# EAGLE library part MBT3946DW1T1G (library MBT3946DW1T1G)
Source: Datasheet
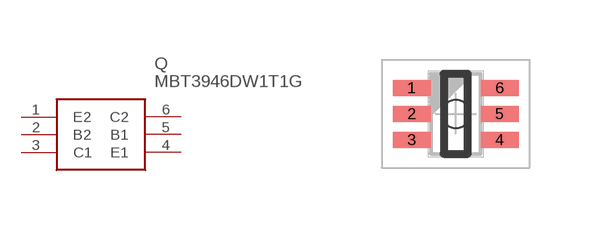
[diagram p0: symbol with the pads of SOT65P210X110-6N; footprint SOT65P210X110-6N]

Designator prefix Q

## MBT3946DW1T1G (Height: 1.1mm; Manufacturer_Name: ON Semiconductor; Manufacturer_Part_Number: MBT3946DW1T1G; Mouser_Part_Number: 863-MBT3946DW1T1G; Mouser_Price-Stock: https://www.mouser.co.uk/ProductDetail/ON-Semiconductor/MBT3946DW1T1G?qs=3JMERSakebo8moNowe%2F%2FpA%3D%3D)  [SOT65P210X110-6N]
1  E2
2  B2
3  C1
4  E1
5  B1
6  C2

## Footprint SOT65P210X110-6N (pad centres in mm)
SC-88(SOT-363) CASE 419B-02
smd 0.95 x 0.4: 1 -1.1,0.65; 2 -1.1,0; 3 -1.1,-0.65; 4 1.1,-0.65; 5 1.1,0; 6 1.1,0.65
